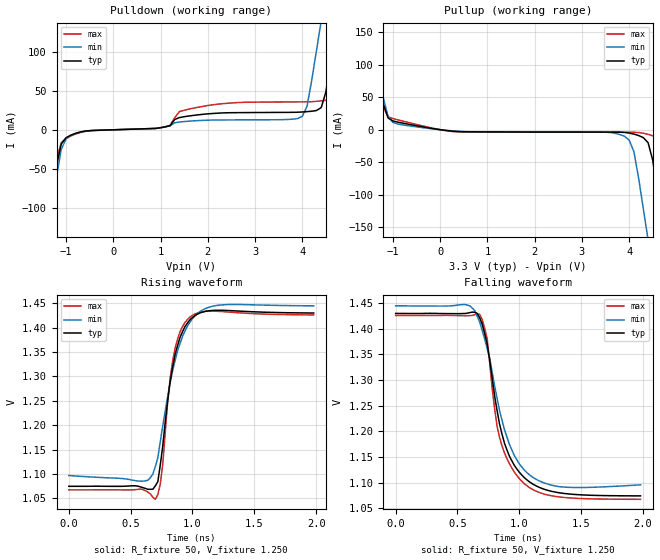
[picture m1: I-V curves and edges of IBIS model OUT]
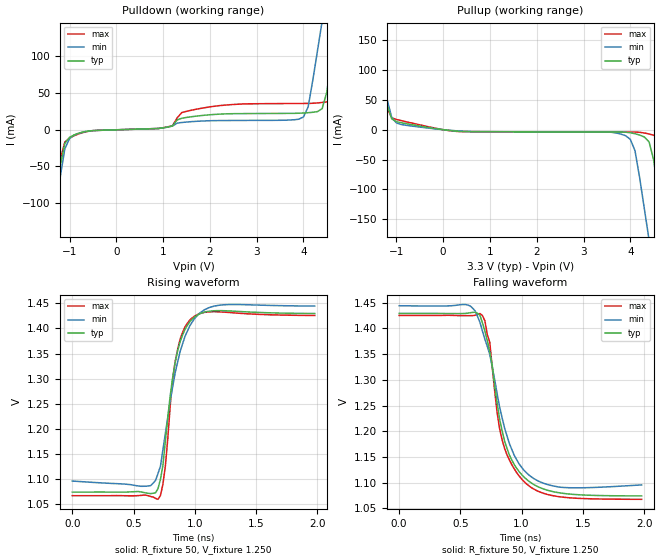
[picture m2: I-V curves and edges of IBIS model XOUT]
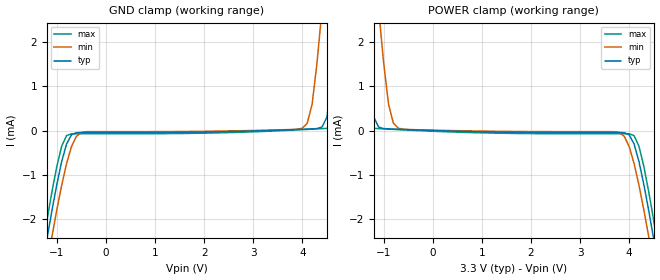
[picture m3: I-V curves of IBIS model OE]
|   IBIS File sg3225van_33v.ibs
[IBIS Ver]   3.2
[File name]   sg3225van_33v.ibs
[File Rev]   1.0
[Date]   May 1, 2013
[Source]
[Disclaimer]
Seiko Epson Corporation makes no warranty with respect to the information
contained herein.
[Copyright]
Copyright(C) 2013, Seiko Epson Corporation. All rights reserved.
|   Component SG3225VAN 3.3V
[Component]   sg3225van_33v
[Manufacturer]   Seiko Epson Corporation
[Package]
R_pkg   0.048   NA   NA
L_pkg   0.48n   NA   NA
C_pkg   0.21p   NA   NA
[Pin] signal_name   model_name   R_pin   L_pin   C_pin
1   OE   OE
2   GND   GND
3   GND   GND
4   OUT   OUT   0.048   0.48n   0.21p
5   XOUT   XOUT   0.048   0.48n   0.21p
6   VCC   POWER
[Diff Pin] inv_pin vdiff   tdelay_typ
4   5   0   0
| Models and submodels in the file (3): OUT (Output), XOUT (Output), OE (Input)
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[Model]   OUT
Model_type Output
Enable Active-High
Polarity Non-Inverting
Vref=1.250
Vmeas=1.250
Rref=50
Cref=0
C_comp   0.12p   0.12p   0.12p
[Temperature Range] 25   105   -40
[Voltage Range]   3.3   2.97   3.63
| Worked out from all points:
|   slope of the pulldown table from 0 to 0.495 V, typ, clamps not added: 507 ohm
|   slope of the pullup table from 0 to 0.495 V, typ, clamps not added: 153 ohm
|   falling waveform, R_fixture 50, V_fixture 1.250: 20-80 % time 186ps typ, 211ps min, 164ps max; typ from 1.43 V to 1.07 V
|   rising waveform, R_fixture 50, V_fixture 1.250: 20-80 % time 121ps typ, 170ps min, 91.2ps max; typ from 1.07 V to 1.43 V
[Pullup]
-3.3V     961.4mA    849mA      1.084A
-1.5V     169.9mA    162.3mA    181mA
-1.2V     39.02mA    48.17mA    34.71mA
-900mV    11.76mA    8.828mA    15.31mA
3.9V      -4.128mA   -10.04mA   -3.846mA
4.1V      -6.665mA   -33.75mA   -3.898mA
4.4V      -19.93mA   -169.4mA   -7.092mA
4.6V      -99.32mA   -264.5mA   -12.36mA
4.7V      -153.1mA   -312mA     -16.55mA
4.8V      -207mA     -359.6mA   -30.08mA
5.1V      -368.7mA   -502.5mA   -197.6mA
6.6V      -1.178A    -1.218A    -1.105A
[Pulldown]
-3.3V     -1.19A     -1.071A    -1.314A
-1.4V     -152.3mA   -155.2mA   -153.8mA
-1.2V     -45.85mA   -59.6mA    -38.08mA
-1.1V     -18.2mA    -25.16mA   -16.54mA
-900mV    -6.981mA   -7.242mA   -8.051mA
3.9V      22.4mA     14.3mA     35.6mA
4.1V      23.13mA    29.95mA    35.69mA
4.4V      28.31mA    139.1mA    36.92mA
4.7V      135mA      252.6mA    39.89mA
4.8V      178.7mA    290.5mA    46.69mA
5V        266.2mA    366.3mA    133.1mA
6.6V      969.2mA    975.5mA    936.7mA
[Falling Waveform]
R_fixture=50
V_fixture=1.250
V_fixture_min=1.271
V_fixture_max=1.238
0s        1.429V     1.444V     1.426V
560ps     1.429V     1.447V     1.425V
680ps     1.421V     1.412V     1.428V
740ps     1.37V      1.361V     1.38V
800ps     1.269V     1.289V     1.244V
840ps     1.214V     1.24V      1.188V
960ps     1.134V     1.153V     1.121V
1.08ns    1.102V     1.116V     1.091V
1.32ns    1.081V     1.092V     1.072V
1.98ns    1.074V     1.096V     1.068V
[Rising Waveform]
R_fixture=50
V_fixture=1.250
V_fixture_min=1.271
V_fixture_max=1.238
0s        1.075V     1.097V     1.067V
600ps     1.072V     1.085V     1.068V
700ps     1.076V     1.115V     1.048V
720ps     1.084V     1.133V     1.057V
740ps     1.119V     1.166V     1.079V
820ps     1.291V     1.287V     1.297V
860ps     1.346V     1.333V     1.359V
980ps     1.416V     1.411V     1.422V
1.2ns     1.436V     1.446V     1.434V
1.98ns    1.43V      1.445V     1.426V
[Ramp]
R_load=50
dV/dt_r   2.133E-1/1.209E-10   2.089E-1/1.701E-10   2.153E-1/9.119E-11
dV/dt_f   2.130E-1/1.860E-10   2.090E-1/2.110E-10   2.147E-1/1.643E-10
|[End   OUT
[Model]   XOUT
Model_type Output
Enable Active-High
Polarity Inverting
Vref=1.250
Vmeas=1.250
Rref=50
Cref=0
C_comp   0.12p   0.12p   0.12p
[Temperature Range] 25   105   -40
[Voltage Range]   3.3   2.97   3.63
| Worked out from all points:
|   slope of the pulldown table from 0 to 0.495 V, typ, clamps not added: 506 ohm
|   slope of the pullup table from 0 to 0.495 V, typ, clamps not added: 153 ohm
|   falling waveform, R_fixture 50, V_fixture 1.250: 20-80 % time 181ps typ, 212ps min, 163ps max; typ from 1.43 V to 1.07 V
|   rising waveform, R_fixture 50, V_fixture 1.250: 20-80 % time 117ps typ, 163ps min, 92.3ps max; typ from 1.07 V to 1.43 V
[Pullup]
-3.3V     1.034A     904mA      1.179A
-1.5V     182.7mA    172.8mA    196.7mA
-1.2V     41.51mA    51.27mA    36.61mA
-900mV    11.8mA     8.855mA    15.37mA
3.9V      -4.132mA   -10.07mA   -3.847mA
4.1V      -6.679mA   -35.39mA   -3.899mA
4.4V      -20.34mA   -184.9mA   -7.112mA
4.6V      -109.6mA   -288.9mA   -12.4mA
4.7V      -169.2mA   -341mA     -16.67mA
4.8V      -228.8mA   -393.1mA   -31.46mA
5.1V      -408.1mA   -549.4mA   -221.2mA
6.6V      -1.305A    -1.332A    -1.239A
[Pulldown]
-3.3V     -1.319A    -1.172A    -1.475A
-1.4V     -168.5mA   -169.6mA   -172.2mA
-1.2V     -49.63mA   -64.75mA   -40.92mA
-1.1V     -18.61mA   -26.05mA   -16.8mA
-900mV    -7.019mA   -7.274mA   -8.114mA
3.9V      22.47mA    14.35mA    35.72mA
4.1V      23.2mA     31.13mA    35.82mA
4.4V      28.75mA    148mA      37.08mA
4.7V      145.1mA    268.8mA    40.16mA
4.8V      192.1mA    309.1mA    48.18mA
5V        286.2mA    389.8mA    144.7mA
6.6V      1.043A     1.039A     1.019A
[Falling Waveform]
R_fixture=50
V_fixture=1.250
V_fixture_min=1.271
V_fixture_max=1.238
0s        1.429V     1.444V     1.425V
560ps     1.43V      1.445V     1.425V
680ps     1.411V     1.395V     1.425V
740ps     1.355V     1.349V     1.373V
800ps     1.255V     1.273V     1.236V
840ps     1.202V     1.227V     1.184V
940ps     1.135V     1.153V     1.127V
1.06ns    1.103V     1.115V     1.094V
1.32ns    1.08V      1.091V     1.072V
1.98ns    1.074V     1.096V     1.068V
[Rising Waveform]
R_fixture=50
V_fixture=1.250
V_fixture_min=1.271
V_fixture_max=1.238
0s        1.074V     1.096V     1.067V
600ps     1.073V     1.086V     1.068V
700ps     1.081V     1.112V     1.06V
760ps     1.176V     1.191V     1.126V
820ps     1.302V     1.284V     1.3V
840ps     1.332V     1.312V     1.334V
920ps     1.398V     1.384V     1.403V
1ns       1.423V     1.42V      1.425V
1.2ns     1.436V     1.446V     1.433V
1.98ns    1.43V      1.445V     1.426V
[Ramp]
R_load=50
dV/dt_r   2.132E-1/1.167E-10   2.089E-1/1.633E-10   2.151E-1/9.226E-11
dV/dt_f   2.129E-1/1.808E-10   2.090E-1/2.120E-10   2.145E-1/1.630E-10
|[End   XOUT
[Model]   OE
Model_type Input
Vinh=2.31
Vinl=0.99
C_comp   3p   3p   3p
[Temperature Range] 25   105   -40
[Voltage Range]   3.3   2.97   3.63
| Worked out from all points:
|   GND clamp passes 1 mA (typ) near -0.96 V on its own axis
|   POWER clamp passes 1 mA (typ) near -1.29 V on its own axis
[GND Clamp]
-3.3V     -17.57mA   -18.04mA   -17.26mA
-1.2V     -2.461mA   -3.05mA    -2.037mA
-900mV    -706.2uA   -1.243mA   -357.4uA
-700mV    -97.47uA   -363.6uA   -75.17uA
4V        28.29uA    52.07uA    20.09uA
4.2V      37.33uA    598uA      31.32uA
4.4V      76.9uA     2.733mA    42.69uA
4.5V      301.4uA    3.927mA    48.43uA
4.7V      2.34mA     6.316mA    64.36uA
4.8V      3.634mA    7.512mA    145.4uA
5.1V      7.519mA    11.1mA     3.362mA
6.6V      27.04mA    29.13mA    24.22mA
[POWER Clamp]
-3.3V     27.04mA    29.13mA    24.22mA
-1.8V     7.519mA    11.1mA     3.362mA
-1.5V     3.634mA    7.512mA    145.4uA
-1.4V     2.34mA     6.316mA    64.36uA
-1.2V     301.4uA    3.927mA    48.43uA
-1.1V     76.9uA     2.733mA    42.69uA
-900mV    37.33uA    598uA      31.32uA
-700mV    28.29uA    52.07uA    20.09uA
4V        -97.47uA   -363.6uA   -75.17uA
4.2V      -706.2uA   -1.243mA   -357.4uA
4.5V      -2.461mA   -3.05mA    -2.036mA
6.6V      -17.57mA   -18.04mA   -17.26mA
